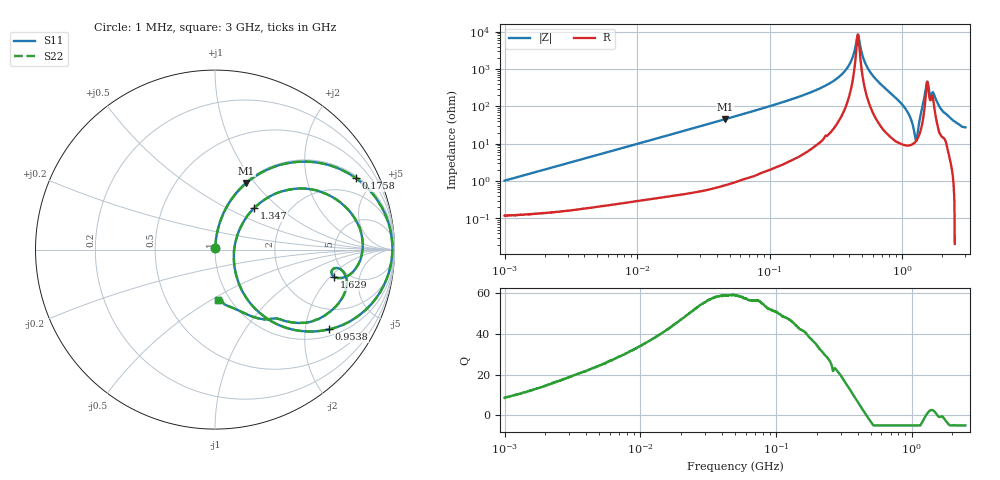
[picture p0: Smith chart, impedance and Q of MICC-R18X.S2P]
!s-Parameter Generated by FASTRON Sdn. Bhd.
!FASTRON P/N : MICC-R18X
!Keysight Technologies,E4991B,MY54100416,A.01.15
!Date: Wed Aug 26 15:55:51 2026
!Version  : Rev00 Wed Aug 26 15:55:51 2026
!Data & Calibration Information:
!PortZ  Port1:50+j0  Port2:50+j0
!When reading, reference impedance value at option line is always used.
! Remarks : This data is being provided solely for informational purposes.
!Freq	S11	S21	S12	S22
# Hz S dB R 50
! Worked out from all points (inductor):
!   1601 points, 1 MHz to 3 GHz, reference 50 ohm
!   read as one part in series: L = 162 nH near 1.041 MHz
!   highest Q = 59.1 at 45.97 MHz (marker M1), where L = 157 nH
!   self-resonance near 461.7 MHz
!   S11 on the Smith chart (normalised r, x): 1 MHz: 1.00, +0.02; 175.8 MHz: 1.10, +3.89; 953.8 MHz: 1.21, -2.70; 1.347 GHz: 1.35, +0.69; 1.629 GHz: 3.93, -2.25; 3 GHz: 0.88, -0.54
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1000000  -39.77 82.8  -0.01 -0.6  -0.01 -0.6  -39.77 82.8
3804036  -28.37 85.1  -0.02 -2.2  -0.02 -2.2  -28.37 85.1
1.447069e7  -17.03 80.5  -0.12 -8.1  -0.12 -8.1  -17.03 80.5
4.597255e7  -7.74 64.8  -0.87 -24.2  -0.87 -24.2  -7.74 64.8
5.477226e7  -6.51 60.8  -1.18 -28.2  -1.18 -28.2  -6.51 60.8
1.757585e8  -1.11 26.9  -6.90 -61.6  -6.90 -61.6  -1.11 26.9
2.083556e8  -0.76 21.9  -8.56 -66.3  -8.56 -66.3  -0.76 21.9
3.631036e8  -0.16 6.8  -18.49 -78.0  -18.49 -78.0  -0.16 6.8
4.114912e8  -0.11 3.4  -24.35 -76.1  -24.35 -76.1  -0.11 3.4
4.639993e8  -0.10 -0.0  -38.65 0.3  -38.65 0.3  -0.10 -0.0
5.583748e8  -0.17 -5.8  -19.84 76.4  -19.84 76.4  -0.17 -5.8
7.925923e8  -0.83 -21.2  -8.82 65.0  -8.82 65.0  -0.83 -21.2
9.538021e8  -2.20 -34.9  -4.83 50.7  -4.83 50.7  -2.20 -34.9
1.125055e9  -6.27 -52.8  -1.88 28.7  -1.88 28.7  -6.27 -52.8
1.262285e9  -18.59 -26.6  -0.95 3.4  -0.95 3.4  -18.59 -26.6
1.347129e9  -9.97 46.7  -1.77 -16.4  -1.77 -16.4  -9.97 46.7
1.423359e9  -4.32 34.0  -4.42 -34.4  -4.42 -34.4  -4.32 34.0
1.503902e9  -1.96 12.5  -11.03 -38.1  -11.03 -38.1  -1.96 12.5
1.629261e9  -3.32 -13.0  -8.67 24.5  -8.67 24.5  -3.32 -13.0
1.921792e9  -4.01 -40.3  -3.60 38.2  -3.60 38.2  -4.01 -40.3
2.383164e9  -7.98 -64.1  -0.91 23.5  -0.91 23.5  -7.98 -64.1
3e9  -11.02 -86.2  0.18 16.0  0.18 16.0  -11.02 -86.2
